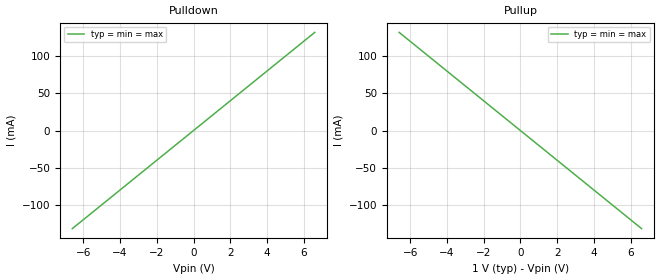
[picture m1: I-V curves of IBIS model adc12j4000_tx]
[IBIS Ver]   5.0
[File Name]   adc12j4000_tx.ibs
[File Rev]   1.0
[Component]   adc12j4000_tx
[Manufacturer] My Company
[Package]
R_pkg  0.0   NA   NA
L_pkg  0.0   NA   NA
C_pkg  0.0   NA   NA
[Pin]   signal_name   model_name   R_pin L_pin  C_pin
1p   adc12j4000_tx_p   adc12j4000_tx
1n   adc12j4000_tx_n   adc12j4000_tx
[Diff_Pin] inv_pin vdiff tdelay_typ tdelay_min tdelay_max
1p   1n   NA   NA   NA   NA
| Models and submodels in the file (1): adc12j4000_tx (Output)
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[Model] adc12j4000_tx
Model_type Output
C_comp 0p 0p 0p
Cref = 0
Vref = 0.5
Rref = 50
Vmeas = 0.5
[Temperature_Range] 25 125 0
[Voltage Range] 1.0 1.0 1.0
[Algorithmic Model]
Executable Windows_cl16.00.40219.01_64 adc12j4000_tx_x64.dll adc12j4000_tx.ami
Executable Windows_cl16.00.40219.01_32 adc12j4000_tx.dll adc12j4000_tx.ami
[End Algorithmic Model]
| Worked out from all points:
|   slope of the pulldown table from 0 to 0.15 V, typ, clamps not added: 50 ohm
|   slope of the pullup table from 0 to 0.15 V, typ, clamps not added: 50 ohm
[Pulldown]
-6.6V     -132mA     -132mA     -132mA
0V        0A         0A         0A
6.6V      132mA      132mA      132mA
[Pullup]
-6.6V     132mA      132mA      132mA
0V        0A         0A         0A
6.6V      -132mA     -132mA     -132mA
[GND Clamp]
-6.6V     0A         0A         0A
0V        0A         0A         0A
6.6V      0A         0A         0A
[Power Clamp]
-6.6V     0A         0A         0A
0V        0A         0A         0A
6.6V      0A         0A         0A
[Ramp]
dV/dt_r 1.0/10p 1.0/10p 1.0/5p
dV/dt_f 1.0/10p 1.0/10p 1.0/5p
